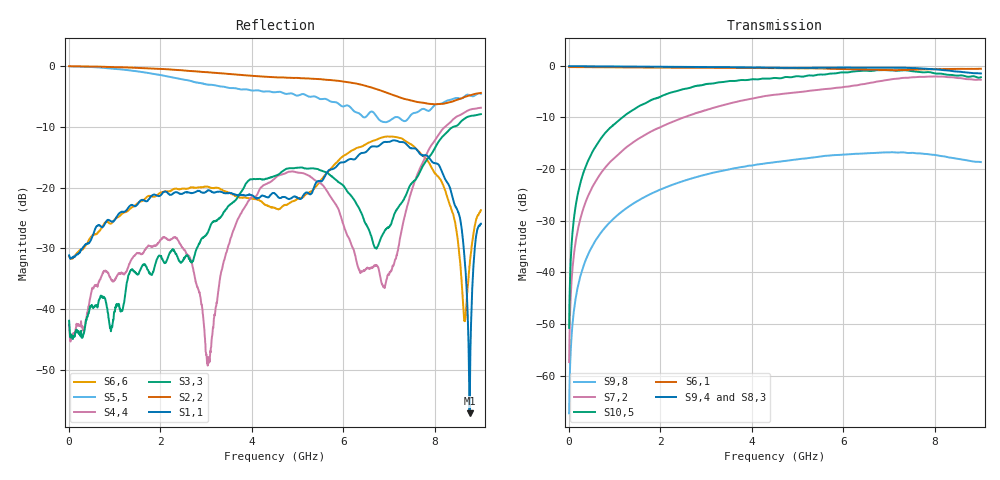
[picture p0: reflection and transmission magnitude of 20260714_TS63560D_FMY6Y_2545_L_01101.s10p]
# GHz S DB R 50
! CMT, SN0916, 25263762, 26.7.0
! Date: 15.07.2026 13:39:49
! Data: Format
! Freq S1.1:dB/Ang S1.2:dB/Ang S1.3:dB/Ang S1.4:dB/Ang S1.5:dB/Ang S1.6:dB/Ang S1.7:dB/Ang S1.8:dB/Ang S1.9:dB/Ang S1.10:dB/Ang
!  S2.1:dB/Ang S2.2:dB/Ang S2.3:dB/Ang S2.4:dB/Ang S2.5:dB/Ang S2.6:dB/Ang S2.7:dB/Ang S2.8:dB/Ang S2.9:dB/Ang S2.10:dB/Ang
!  S3.1:dB/Ang S3.2:dB/Ang S3.3:dB/Ang S3.4:dB/Ang S3.5:dB/Ang S3.6:dB/Ang S3.7:dB/Ang S3.8:dB/Ang S3.9:dB/Ang S3.10:dB/Ang
!  S4.1:dB/Ang S4.2:dB/Ang S4.3:dB/Ang S4.4:dB/Ang S4.5:dB/Ang S4.6:dB/Ang S4.7:dB/Ang S4.8:dB/Ang S4.9:dB/Ang S4.10:dB/Ang
!  S5.1:dB/Ang S5.2:dB/Ang S5.3:dB/Ang S5.4:dB/Ang S5.5:dB/Ang S5.6:dB/Ang S5.7:dB/Ang S5.8:dB/Ang S5.9:dB/Ang S5.10:dB/Ang
!  S6.1:dB/Ang S6.2:dB/Ang S6.3:dB/Ang S6.4:dB/Ang S6.5:dB/Ang S6.6:dB/Ang S6.7:dB/Ang S6.8:dB/Ang S6.9:dB/Ang S6.10:dB/Ang
!  S7.1:dB/Ang S7.2:dB/Ang S7.3:dB/Ang S7.4:dB/Ang S7.5:dB/Ang S7.6:dB/Ang S7.7:dB/Ang S7.8:dB/Ang S7.9:dB/Ang S7.10:dB/Ang
!  S8.1:dB/Ang S8.2:dB/Ang S8.3:dB/Ang S8.4:dB/Ang S8.5:dB/Ang S8.6:dB/Ang S8.7:dB/Ang S8.8:dB/Ang S8.9:dB/Ang S8.10:dB/Ang
!  S9.1:dB/Ang S9.2:dB/Ang S9.3:dB/Ang S9.4:dB/Ang S9.5:dB/Ang S9.6:dB/Ang S9.7:dB/Ang S9.8:dB/Ang S9.9:dB/Ang S9.10:dB/Ang
!  S10.1:dB/Ang S10.2:dB/Ang S10.3:dB/Ang S10.4:dB/Ang S10.5:dB/Ang S10.6:dB/Ang S10.7:dB/Ang S10.8:dB/Ang S10.9:dB/Ang S10.10:dB/Ang
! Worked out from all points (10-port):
!   2001 points, 10 MHz to 9 GHz, reference 50 ohm
!   strongest paths, dB at 10 MHz, 2.257 GHz, 4.505 GHz, 6.753 GHz, 9 GHz:
!     S9,4: -0.1, -0.2, -0.4, -0.4, -1.5
!     S8,3: -0.1, -0.2, -0.4, -0.4, -1.3
!     S6,1: -0.3, -0.4, -0.5, -0.8, -0.6
!     S10,5: -50.8, -5.1, -2.4, -0.8, -2.2
!     S7,2: -57.4, -10.9, -5.6, -3.0, -2.7
!     S9,8: -67.3, -23.1, -18.7, -16.8, -18.6
!   lowest |S11| = -57.1 dB at 8.753 GHz (marker M1), VSWR 1.00, Z = 50 - j0.139 ohm
!   |S11| at or under -10 dB: start of sweep to end of sweep
